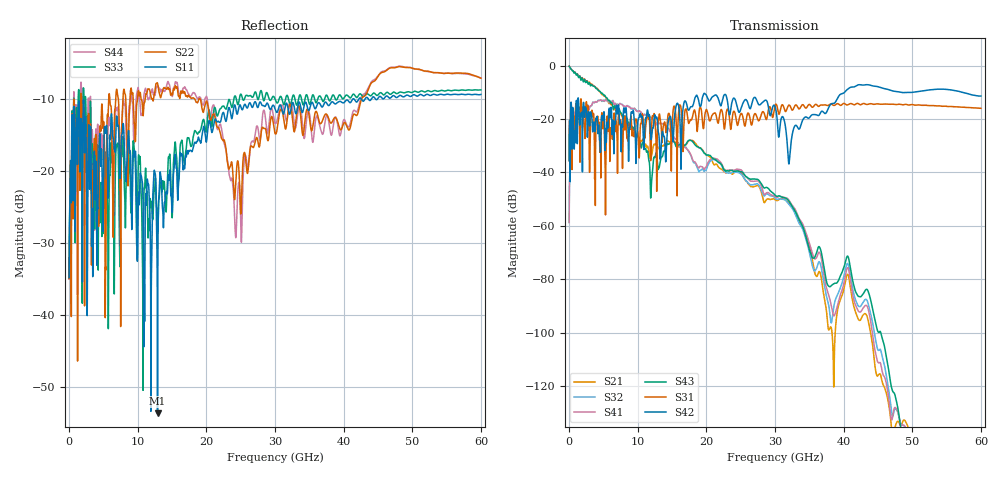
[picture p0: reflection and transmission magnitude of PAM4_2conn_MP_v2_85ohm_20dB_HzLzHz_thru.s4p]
! Info: Touchstone file created by Circ.  Input file=FAB50GbE_2conn_Midplane_Examax_Topo2_v2_85ohm_20dB_HzLzHz.circ
# Hz S RI R 50
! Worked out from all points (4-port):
!   6000 points, 10 MHz to 60 GHz, reference 50 ohm
!   strongest paths, dB at 10 MHz, 15.01 GHz, 30.01 GHz, 45.01 GHz, 60 GHz:
!     S42: -35.5, -24.0, -15.3, -7.9, -11.4
!     S31: -35.6, -23.2, -14.9, -14.3, -16.0
!     S43: -0.2, -27.6, -48.5, -99.7, -162.7
!     S41: -58.7, -26.0, -49.1, -111.1, -161.6
!     S32: -58.7, -26.1, -49.6, -106.5, -156.5
!     S21: -0.2, -27.8, -50.2, -116.0, -153.7
!   lowest |S11| = -53.6 dB at 12.89 GHz (marker M1), VSWR 1.00, Z = 50.2 - j0.0211 ohm
!   |S11| at or under -10 dB: start of sweep to 41.32 GHz; 41.55 GHz to 42.2 GHz (645.9 MHz wide, 1.54 % of centre); 42.59 GHz to 43.11 GHz (522.1 MHz wide, 1.22 % of centre)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
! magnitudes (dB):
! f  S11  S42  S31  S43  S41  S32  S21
! 10 MHz  -34.8  -35.5  -35.6  -0.2  -58.7  -58.7  -0.2
! 1.13 GHz  -13.1  -14.7  -16.6  -3.4  -19.8  -20.0  -3.2
! 12.89 GHz  -53.6  -21.3  -23.2  -37.0  -22.1  -22.2  -30.3
! 24.26 GHz  -11.1  -13.1  -18.8  -39.5  -38.9  -39.9  -39.6
! 31.64 GHz  -10.6  -25.2  -16.9  -49.7  -49.5  -50.7  -50.5
! 37.3 GHz  -10.4  -17.9  -14.7  -78.0  -81.0  -83.8  -88.6
! 60 GHz  -9.3  -11.4  -16.0  -162.7  -161.6  -156.5  -153.7
